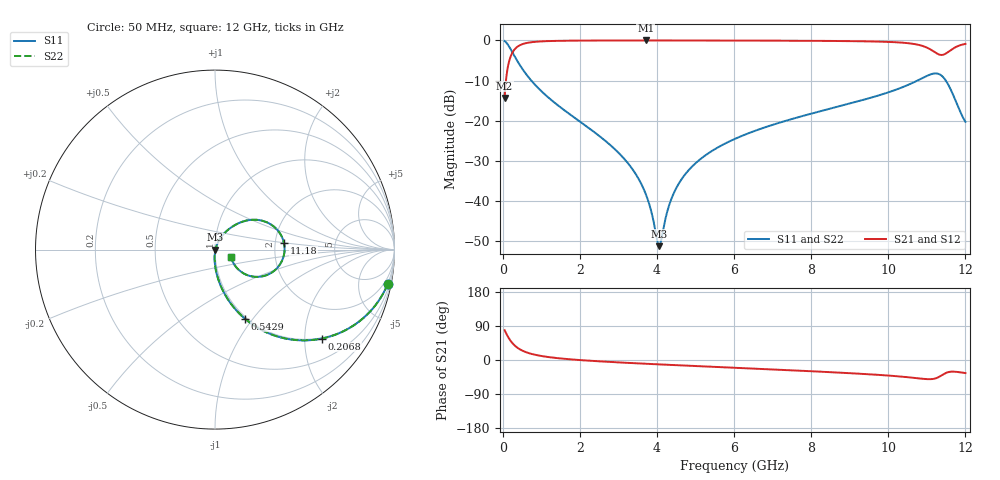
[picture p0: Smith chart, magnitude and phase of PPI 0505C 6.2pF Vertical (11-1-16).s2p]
# GHz S MA R 50
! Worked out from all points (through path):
!   1601 points, 50 MHz to 12 GHz, reference 50 ohm
!   highest |S21| = -0.03 dB at 3.71 GHz (marker M1); lowest = -14.3 dB at 50 MHz (marker M2)
!   group delay of S21, straight-line fit = 15.6 ps
!   lowest |S11| = -51.3 dB at 4.061 GHz (marker M3), VSWR 1.01, Z = 50.3 - j0.0475 ohm
!   |S11| at or under -10 dB: 740.8 MHz to 10.76 GHz (10.02 GHz wide, 174 % of centre); 11.49 GHz to end of sweep
!   |S22| runs from -51.3 to -0.2 dB; largest |S21 - S12| = 0
!   S11 on the Smith chart (normalised r, x): 50 MHz: 1, -10; 206.8 MHz: 0.98, -2.43; 542.9 MHz: 0.98, -0.91; 11.18 GHz: 2.24, +0.19; 12 GHz: 1.19, -0.09
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0.05  0.9813 -11.2  0.1923 78.8  0.1923 78.8  0.9813 -11.2
0.139625  0.8769 -29.1  0.4803 60.9  0.4803 60.9  0.8769 -29.1
0.2068437  0.7758 -39.7  0.6304 50.3  0.6304 50.3  0.7758 -39.7
0.3562187  0.5792 -55.5  0.8144 34.4  0.8144 34.4  0.5792 -55.5
0.5429375  0.4191 -66.6  0.9068 23.2  0.9068 23.2  0.4191 -66.6
1.020938  0.2286 -79.4  0.972 10.3  0.972 10.3  0.2286 -79.4
2.044156  0.09422 -89.3  0.9935 -0.5  0.9935 -0.5  0.09422 -89.3
3.134594  0.0342 -93.0  0.9968 -7.0  0.9968 -7.0  0.0342 -93.0
3.470687  0.02087 -91.8  0.997 -8.7  0.997 -8.7  0.02087 -91.8
3.709687  0.01223 -87.6  0.9971 -9.9  0.9971 -9.9  0.01223 -87.6
4.038312  0.002805 -25.2  0.997 -11.5  0.997 -11.5  0.002805 -25.2
4.060719  0.002735 -9.9  0.997 -11.6  0.997 -11.6  0.002735 -9.9
4.359469  0.01014 60.7  0.9968 -13.0  0.9968 -13.0  0.01014 60.7
4.680625  0.0199 67.0  0.9965 -14.5  0.9965 -14.5  0.0199 67.0
5.225844  0.03608 68.0  0.9958 -17.0  0.9958 -17.0  0.03608 68.0
6.025  0.05937 66.1  0.9943 -20.5  0.9943 -20.5  0.05937 66.1
8.019156  0.1229 57.9  0.9867 -29.7  0.9867 -29.7  0.1229 57.9
10.01331  0.2261 44.4  0.956 -41.1  0.956 -41.1  0.2261 44.4
10.79753  0.3228 28.5  0.8763 -48.6  0.8763 -48.6  0.3228 28.5
11.17844  0.3859 5.5  0.7274 -49.7  0.7274 -49.7  0.3859 5.5
11.52947  0.2954 -30.7  0.704 -32.8  0.704 -32.8  0.2954 -30.7
12  0.09684 -23.7  0.9039 -34.4  0.9039 -34.4  0.09684 -23.7
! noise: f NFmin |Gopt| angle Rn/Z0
0.05  0.0005387  0.9066  1.652  0.001266
1.372  0.004814  0.7226  4.446  0.003436
2.701  0.00786  0.675  7.984  0.004642
4.031  0.01062  0.6478  11.53  0.005668
5.36  0.01337  0.6326  15.03  0.006728
6.682  0.0164  0.6292  18.47  0.008095
8.012  0.02064  0.6453  21.95  0.01064
9.341  0.02991  0.706  25.63  0.01903
10.67  0.07769  0.8599  29.65  0.111
12  0.1096  0.8873  33.4  0.1939
